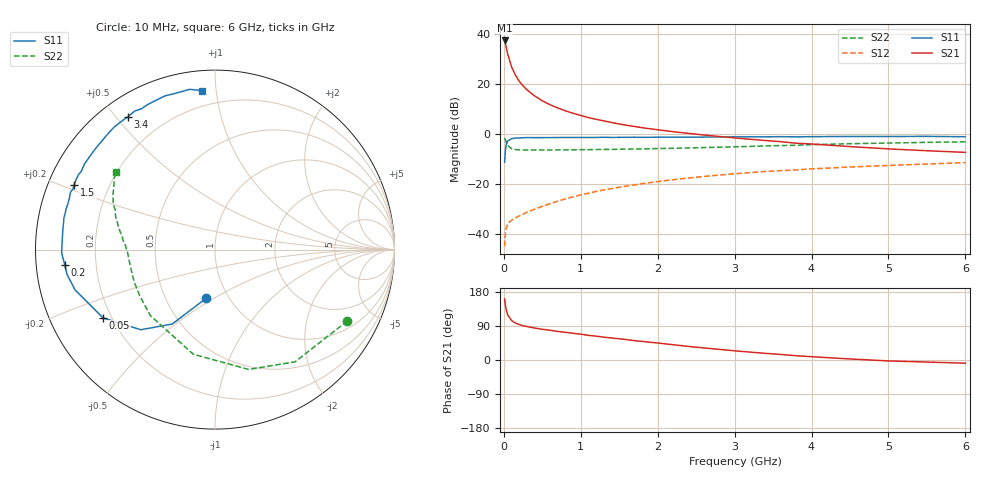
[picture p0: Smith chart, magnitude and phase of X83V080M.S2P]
! SIEMENS Small Signal Semiconductors
! BFP136W
! Si NPN RF Bipolar Junction Transistor in SOT343
! VCE = 3 V  IC = 80 mA
! Common Emitter S-Parameters:  September  1994
# GHz  S  MA  R  50
!  f  S11  S21  S12  S22
! GHz  MAG  ANG  MAG  ANG  MAG  ANG  MAG  ANG
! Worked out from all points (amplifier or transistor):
!   40 points, 10 MHz to 6 GHz, reference 50 ohm
!   highest |S21| = 37.6 dB at 10 MHz (marker M1)
!   |S21| within 3 dB of that: start of sweep to 32.63 MHz
!   unconditionally stable (mu >= 1): 553.9 MHz to 2.875 GHz
!   at 200 MHz: K = 0.65, MSG = 27.0 dB, |S12| = -32.7 dB
!   at 1.5 GHz: K = 1.10, MAG = 10.7 dB, |S12| = -21.3 dB
!   at 6 GHz: K = 0.97, MSG = 2.1 dB, |S12| = -11.4 dB
!   S11 on the Smith chart (normalised r, x): 10 MHz: 0.79, -0.46; 50 MHz: 0.17, -0.27; 200 MHz: 0.09, -0.05; 1.5 GHz: 0.08, +0.22; 3.4 GHz: 0.08, +0.54; 6 GHz: 0.11, +0.92
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0.01  0.2738 -100.0  75.53 161.0  0.0057 69.4  0.8379 -28.3
0.02  0.4784 -119.9  65.58 145.0  0.01 59.8  0.7681 -54.5
0.03  0.6085 -132.8  55.81 133.5  0.013 50.7  0.6936 -74.3
0.05  0.7305 -148.6  40.27 119.1  0.016 39.4  0.5955 -101.7
0.1  0.8112 -163.9  22.44 104.2  0.0188 35.2  0.5146 -134.5
0.15  0.8361 -170.5  15.3 97.5  0.0209 37.5  0.4919 -148.5
0.2  0.8408 -174.1  11.5 93.5  0.0231 39.8  0.4854 -156.2
0.25  0.849 -177.0  9.278 90.5  0.025 42.5  0.483 -161.0
0.3  0.8548 -178.9  7.765 88.3  0.0273 45.0  0.4806 -164.3
0.4  0.8527 177.4  5.847 84.4  0.0315 49.0  0.4808 -168.7
0.5  0.8533 174.6  4.663 81.1  0.0359 52.3  0.4815 -171.6
0.6  0.8549 172.7  3.892 78.5  0.0404 54.6  0.4825 -173.6
0.7  0.8569 169.9  3.354 75.4  0.0453 57.3  0.4838 -174.9
0.9  0.8587 166.5  2.624 70.4  0.0555 58.5  0.4863 -177.5
1.1  0.8584 162.1  2.149 65.0  0.0658 59.7  0.4903 -179.2
1.5  0.8632 155.5  1.6 56.0  0.0865 59.3  0.4982 177.8
2.2  0.8697 143.1  1.122 40.3  0.1224 54.9  0.5206 172.4
3.2  0.8845 126.1  0.79 20.8  0.1695 45.8  0.5689 163.7
3.4  0.8854 123.3  0.747 17.5  0.1792 43.8  0.5826 161.8
4.5  0.9007 108.1  0.564 2.8  0.2196 33.7  0.6444 151.9
5.5  0.9041 99.0  0.466 -5.4  0.2525 25.9  0.6862 144.9
6  0.8883 94.6  0.432 -8.4  0.2693 21.5  0.7026 141.9
